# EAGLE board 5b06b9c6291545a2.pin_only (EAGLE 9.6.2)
REV: C

Size 50.8 x 22.86 mm. Coordinates in mm from the lower left corner, seen from the top.
Outline: 2.54,0 48.26,0 arc90 50.8,2.54 50.8,20.32 arc90 48.26,22.86 2.54,22.86 arc90 0,20.32 0,2.54 arc90 2.54,0
Copper layers (1*16): Top 0.035mm / dielectric 1.5mm / Bottom 0.035mm
Design rules "adafruit 7-7 *": minimum track width 6mil, minimum drill 15.5mil, track to track 8mil, track to pad 7mil, pad to pad 7mil, via to via 7mil, smd to smd 7mil, copper to edge 10mil, drill to drill 8mil, minimum pad ring 10mil, minimum via ring 8mil, stop-mask expansion 2mil, vias tented up to drill 20mil, thermal gap 10mil
Net classes: 2 gnd: width 0.254 mm, drill 0.483 mm; 3 Power: width 0.305 mm, drill 0.483 mm
Holes 2.2 mm at 48.26,1.84 48.26,20.95

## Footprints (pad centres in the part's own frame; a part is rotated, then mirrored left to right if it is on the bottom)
0805-NO = smd 1.24 x 1.5: 1 -0.95,0; 2 0.95,0
0603-NO = smd 1.075 x 1: 1 -0.85,0; 2 0.85,0
_0805MP = smd 1.2 x 1.3: 1 -1.016,0; 2 1.016,0
CHIPLED_0603_NOOUTLINE = smd 0.8 x 0.8: A 0,-0.75; C 0,0.75
JST_SH4_RA = smd 0.6 x 1.55: 1 1.5,1.686; 2 0.5,1.686; 3 -0.5,1.686; 4 -1.5,1.686 | smd 1.2 x 1.8: MT1 -2.8,-0.862; MT2 2.8,-0.862
SOD-123 = smd 1.4 x 1.4: A 1.85,0; C -1.85,0
WLCSP9 = smd 0.275 x 0.275: A1 -0.5,0.5; A2 0,0.5; A3 0.5,0.5; B1 -0.5,0; B2 0,0; B3 0.5,0; C1 -0.5,-0.5; C2 0,-0.5; C3 0.5,-0.5
1X16_ROUND = drill 1 pad 1.676: 1 -19.05,0; 2 -16.51,0; 3 -13.97,0; 4 -11.43,0; 5 -8.89,0; 6 -6.35,0; 7 -3.81,0; 8 -1.27,0; 9 1.27,0; 10 3.81,0; 11 6.35,0; 12 8.89,0; 13 11.43,0; 14 13.97,0; 15 16.51,0; 16 19.05,0
1X12_ROUND = drill 1 pad 1.676: 1 -13.97,0; 2 -11.43,0; 3 -8.89,0; 4 -6.35,0; 5 -3.81,0; 6 -1.27,0; 7 1.27,0; 8 3.81,0; 9 6.35,0; 10 8.89,0; 11 11.43,0; 12 13.97,0
SK6805_1515 = smd 0.5 x 0.5: 1 -0.5,-0.45; 2 0.5,-0.45; 3 0.5,0.45; 4 -0.5,0.45
SOT23-R = smd 0.635 x 1.016: 1 -0.95,-1; 2 0.95,-1; 3 0,1
RESPACK_4X0603 = smd 0.45 x 0.9: 1 -1.3,-0.85; 2 -0.4,-0.85; 3 0.4,-0.85; 4 1.3,-0.85; 5 1.3,0.85; 6 0.4,0.85; 7 -0.4,0.85; 8 -1.3,0.85
BTN_KMR2_4.6X2.8 = smd 0.9 x 0.9: A 2.05,0.8; A' -2.05,0.8; B 2.05,-0.8; B' -2.05,-0.8
TESTPOINT_ROUND_1.5MM_NO = smd 1.5 x 1.5: P$1 0,0
QFN60_ESP32-S2-MINI-1_EXP = smd 0.813 x 0.406: 1 -7,3.645; 2 -7,2.795; 3 -7,1.945; 4 -7,1.095; 5 -7,0.245; 6 -7,-0.605; 7 -7,-1.455; 8 -7,-2.305; 9 -7,-3.155; 10 -7,-4.005; 11 -7,-4.855; 12 -7,-5.705; 13 -7,-6.555; 14 -7,-7.405; 15 -7,-8.255; 31 7,-8.255; 32 7,-7.405; 33 7,-6.555; 34 7,-5.705; 35 7,-4.855; 36 7,-4.005; 37 7,-3.155; 38 7,-2.305; 39 7,-1.455; 40 7,-0.605; 41 7,0.245; 42 7,1.095; 43 7,1.945; 44 7,2.795; 45 7,3.645 | smd 0.406 x 0.813: 16 -5.95,-9.305; 17 -5.1,-9.305; 18 -4.25,-9.305; 19 -3.4,-9.305; 20 -2.55,-9.305; 21 -1.7,-9.305; 22 -0.85,-9.305; 23 0,-9.305; 24 0.85,-9.305; 25 1.7,-9.305; 26 2.55,-9.305; 27 3.4,-9.305; 28 4.25,-9.305; 29 5.1,-9.305; 30 5.95,-9.305; 46 5.95,4.695; 47 5.1,4.695; 48 4.25,4.695; 49 3.4,4.695; 50 2.55,4.695; 51 1.7,4.695; 52 0.85,4.695; 53 0,4.695; 54 -0.85,4.695; 55 -1.7,4.695; 56 -2.55,4.695; 57 -3.4,4.695; 58 -4.25,4.695; 59 -5.1,4.695; 60 -5.95,4.695 | smd 1.194 x 1.194: 61 0,-2.305; 66 -1.65,-0.655; 67 0,-0.655; 68 1.65,-0.655; 69 -1.65,-2.305; 70 1.65,-2.305; 71 -1.65,-3.955; 72 0,-3.955; 73 1.65,-3.955 | smd 0.813 x 0.813: 62 -7,4.695; 63 -7,-9.305; 64 7,-9.305; 65 7,4.695
SOT23-5 = smd 0.55 x 1.2: 1 -0.95,-1.3; 2 0,-1.3; 3 0.95,-1.3; 4 0.95,1.3; 5 -0.95,1.3
BME280 = smd 0.5 x 0.35: 1 1.025,0.975; 2 1.025,0.325; 3 1.025,-0.325; 4 1.025,-0.975; 5 -1.025,-0.975; 6 -1.025,-0.325; 7 -1.025,0.325; 8 -1.025,0.975
MOUNTINGHOLE_2.5_PLATED = drill 2.5 pad 3.2: P$1 0,0
FIDUCIAL_1MM = smd 1 x 1: 1 0,0
JSTPH2_BATT = smd 1 x 4.6: 1 -1,-3.7; 2 1,-3.7 | smd 1.6 x 3.4: NC1 -3.4,1.5; NC2 3.4,1.5
USB_C_CUSB31-CFM2AX-01-X = smd 0.575 x 1.15: A1B12 -3.2,3.545; A4B9 -2.4,3.545; B1A12 3.2,3.545; B4A9 2.4,3.545 | smd 0.275 x 1.15: A5 -1.25,3.545; A6 -0.25,3.545; A7 0.25,3.545; A8 1.25,3.545; B5 1.75,3.545; B6 0.75,3.545; B7 -0.75,3.545; B8 -1.75,3.545 | drill 0.6 pad 1 long: M1 -4.32,2.97; M2 4.32,2.97; M3 -4.32,-1.21; M4 4.32,-1.21 | hole 0.65: 2.89,2.47; -2.89,2.47

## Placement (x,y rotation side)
C1  10uF  [0805-NO]  15.94,13.13 0 top
C2  10uF  [0805-NO]  18.66,11.94 90 top
C3  10µF  [0805-NO]  21.54,16 0 top
C4  1uF  [0603-NO]  14.17,5.28 90 top
C5  1uF  [0603-NO]  28.77,4 180 top
C6  10µF  [0805-NO]  12.94,9.39 270 top
C7  10uF  [0805-NO]  28.07,17.84 0 top
C8  10µF  [0805-NO]  17.34,5.45 270 top
C9  10uF  [0805-NO]  28.07,15.94 0 top
C10  1uF  [0603-NO]  44.58,19.81 0 top
C11  10uF  [_0805MP]  26.04,8.51 0 top
CHG  ORANGE  [CHIPLED_0603_NOOUTLINE]  1.46,5.46 270 top
CONN1  JST SH  [JST_SH4_RA]  22.35,11.43 270 top
D3  RED  [CHIPLED_0603_NOOUTLINE]  1.46,17.53 90 top
D4  MBR540  [SOD-123]  11.48,11.99 180 top
IC1  LC709203F/MH  [WLCSP9]  21.84,18.03 90 top
JP1  [1X16_ROUND]  25.4,1.27 180 top
JP3  [1X12_ROUND]  30.48,21.59 0 top
LED1  WS2812B_SK6805_1515  [SK6805_1515]  29.4,8.13 0 top
Q3  DMG3415U  [SOT23-R]  10.4,9.51 0 top
R1  5.1K  [0603-NO]  15.75,5.33 90 top
R2  5.1K  [0603-NO]  6.34,4.11 0 top
R3  10K  [RESPACK_4X0603]  26.92,11.94 270 top
R4  5.1K  [0603-NO]  15.67,15.88 90 top
R5  5.1K  [0603-NO]  8.19,8.28 90 top
R7  100K  [0603-NO]  18.67,8.88 0 top
R8  5.1K  [0603-NO]  5.08,17.27 0 top
R10  5.1K  [0603-NO]  5.71,20.45 270 top
R12  100K  [0603-NO]  6.36,5.66 180 top
R17  1Meg  [0603-NO]  28.77,5.52 0 top
SW1  KMR2  [BTN_KMR2_4.6X2.8]  20.95,5.21 0 top
SW2  KMR2  [BTN_KMR2_4.6X2.8]  10.79,5.14 0 top
TP1  [TESTPOINT_ROUND_1.5MM_NO]  20.45,5.41 0 bottom
U1  ESP32-S3-MINI-1  [QFN60_ESP32-S2-MINI-1_EXP]  40.64,11.43 270 top
U2  AP2112/RT9080-3.3  [SOT23-5]  15.54,10.16 0 top
U3  MCP73831T-2ACI/OT  [SOT23-5]  18.11,16.26 0 top
U4  BME280  [BME280]  24.77,16 90 top
U5  AP2112/RT9080-3.3  [SOT23-5]  25.53,5.59 0 top
U$14  [PCBFEAT-REV-040]  25.27,12.26 0 bottom
U$15  [FEATHERLOGO_MED]  23.88,6.6 0 bottom
U$31  MOUNTINGHOLE2.5  [MOUNTINGHOLE_2.5_PLATED]  2.54,20.32 270 top
U$32  MOUNTINGHOLE2.5  [MOUNTINGHOLE_2.5_PLATED]  2.54,2.54 270 top
U$34  FIDUCIAL_1MM  [FIDUCIAL_1MM]  11.43,21.08 270 top
U$35  FIDUCIAL_1MM  [FIDUCIAL_1MM]  46.38,1 270 top
U$53  [STEMMAQT]  21.34,11.18 0 bottom
X1  JSTPH  [JSTPH2_BATT]  10.92,19.37 0 top
X3  USB C  [USB_C_CUSB31-CFM2AX-01-X]  2.67,11.43 270 top

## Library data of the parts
C1-C7 C9-C11 CHG CONN1 D3 D4 JP1 JP3 LED1 Q3 R1-R5 R7 R8 R10 R12 R17 SW1 SW2 TP1 U2 U3 U5 = microbuilder
C8 = microbuilder; COMPANY: ADAFRUIT INDUSTRIES; DRAWN: KTOWN; REV: C
IC1 U4 = adafruit_sensor
U1 = adafruit_wireless; BUILT_BY: EMA_Kyle; COPYRIGHT: Copyright (C) 2018 Accelerated Designs. All rights reserved; DATASHEET: https://www.espressif.com/sites/default/files/documentation/esp32-s2-mini-1_esp32-s2-mini-1u_datasheet_en.pdf; MANUFACTURER_PART_NUMBER: ESP32-S2-MINI-1; SOURCELIBRARY: Add_to_database_2020-11-03; VENDOR: Espressif Systems
U$14 = microbuilder; REV: C
U$15 = feather_silks
U$31 U$32 U$34 U$35 = microbuilder; BOM: EXCLUDE
U$53 = silks
X1 = adafruit_electromech
X3 = adafruit_connector

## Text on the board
tPlace: SDA | BAT | EN | USB | 13 | 12 | 11 | 10 | 9 | 6 | 5 | SCL | #13 | I2C | ESP32S3 | Reset | Boot | Neo | Chg | RST | 3V | 3V | GND | A0 | A1 | A2 | A3 | A4 | A5 | SCK | MO | MI | RX | TX | DB
bPlace: 3.7/4.2V / LiPoly Batt / µUSB charge | EN | 13 | 12 | 11 | 10 | 9 | 6 | 5 | BAT | USB | SCL | SDA | ESP32-S3 Feather / 240MHz Tensilica / WiFi Microcontroller / 8M Flash No PSRAM | RST | GND | SCK | 3V | 3V | A0 | A1 | A2 | A3 | A4 | A5 | MO | MI | RX | TX | Debug / TX

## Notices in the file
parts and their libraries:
microbuilder: This work is placed in the public domain, and may be freely used for commercial and non-commercial work with the following conditions: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
